FUNCTION_BLOCK FB_Blinker
VAR_INPUT
	CLK: BOOL;
END_VAR
VAR_OUTPUT
	Q: BOOL;
END_VAR
VAR
	fbTimer1: TON;
	fbTimer2: TON;
END_VAR

fbTimer1(IN :=(NOT fbTimer2.Q AND CLK), PT := T#1S);
fbTimer2(IN := fbTimer1.Q, PT := T#1S);
Q := fbTimer1.Q;

END_FUNCTION_BLOCK
